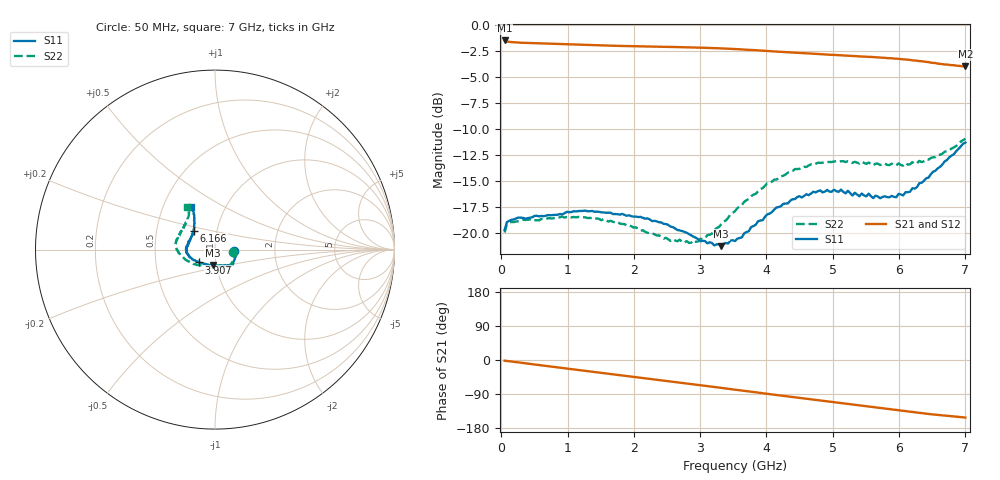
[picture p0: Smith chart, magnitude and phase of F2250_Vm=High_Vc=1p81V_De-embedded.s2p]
! Integrated Device Technology
! Corporate Headquarters
! 6024 Silver Creek Valley Road
! San Jose, CA 95138  USA
! Phone:  1-408-284-8200
! Toll Free:  1-800-223-1366
! Webpage:  http://www.idt.com/
! Timing and RF Division
! 515 Groton Road, Suite 102
! Westford, MA 01886-6024
! Device:  F2250
! Description: Voltage Variable RF Attenuator
! Frequency:  50.0 -  6000.00 MHz
! Package:  3x3 mm Thin QFN Plastic Package: 16 pin
! Ports:  2 RF, 3 DC
!  Pin  1  = GND
!  Pin  2  = NC
!  Pin  3  = RF1  = Port 1
!  Pin  4  = NC
!  Pin  5  = GND
!  Pin  6  = GND
!  Pin  7  = GND
!  Pin  8  = GND
!  Pin  9  = NC
!  Pin 10  = RF2  = Port 2
!  Pin 11  = NC
!  Pin 12  = GND
!  Pin 13  = GND
!  Pin 14  = VCNTRL
!  Pin 15  = VDD
!  Pin 16  = VMODE
! Vcntrl:  1.810 Volts
! Vmode:  +3.300 Volts
! Vdd:  +3.30  Volts
! Current:  1.324 mA
! Data:  The device was measured on a the F2250 evaluation board which has
!  individual transmission lines to the RF pins.  Data was collected
!  using a calibrated network analyzer.  The evaluation board was
!  de-embedded using a TRL calibration technique.
!  The reference plane is the edge of the package pin.
! Misc:  SN 10
!  Action Tracker AT0258
! Date Measured:  2014-11-26
! Date:  2015-10-15  MJV
! Note:
!  Integrated Device Technology supplies this data as a sample of measured
!  data at the package pin for this product.  Your particular data for this
!  product may vary.
!  Data was taken at 25 degrees C.
!  Integrated Device Technology reserves the right to change this data at anytime.
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# GHz S dB R 50
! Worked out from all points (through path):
!   201 points, 50 MHz to 7 GHz, reference 50 ohm
!   highest |S21| = -1.46 dB at 50 MHz (marker M1); lowest = -4.0 dB at 7 GHz (marker M2)
!   group delay of S21, straight-line fit = 61 ps
!   lowest |S11| = -21.2 dB at 3.317 GHz (marker M3), VSWR 1.19, Z = 48.2 - j8.35 ohm
!   |S11| at or under -10 dB: start of sweep to end of sweep
!   |S22| runs from -20.9 to -10.9 dB; largest |S21 - S12| = 0.0018
!   S11 on the Smith chart (normalised r, x): 50 MHz: 1.23, -0.02; 3.907 GHz: 0.83, -0.12; 6.166 GHz: 0.77, +0.17; 7 GHz: 0.69, +0.36
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0.05  -19.67 -5.2  -1.46 -1.9  -1.46 -1.8  -19.92 -6.5
0.08475  -18.91 -5.1  -1.57 -2.5  -1.56 -2.5  -19.11 -6.2
0.1195  -18.80 -5.9  -1.60 -3.3  -1.60 -3.3  -18.94 -6.3
0.6755  -18.29 -25.0  -1.75 -15.7  -1.75 -15.7  -18.62 -29.6
1.2315  -17.84 -40.9  -1.88 -27.9  -1.89 -27.9  -18.44 -50.9
1.75275  -18.16 -47.9  -1.98 -39.1  -1.98 -39.1  -18.88 -61.6
2.37825  -18.93 -51.2  -2.07 -52.6  -2.07 -52.6  -20.19 -72.4
2.552  -19.35 -54.5  -2.08 -56.4  -2.08 -56.4  -20.72 -78.9
2.86475  -20.18 -64.1  -2.13 -63.4  -2.13 -63.4  -20.90 -94.8
3.07325  -20.75 -76.6  -2.17 -68.1  -2.17 -68.1  -20.45 -109.2
3.3165  -21.23 -97.5  -2.23 -73.7  -2.23 -73.7  -19.15 -126.0
3.525  -20.74 -115.5  -2.29 -78.4  -2.29 -78.4  -17.87 -138.0
3.90725  -18.77 -141.4  -2.43 -87.0  -2.43 -87.0  -15.74 -156.4
4.1505  -17.51 -153.8  -2.53 -92.4  -2.53 -92.5  -14.83 -165.8
4.4285  -16.70 -163.8  -2.64 -98.5  -2.64 -98.6  -13.83 -174.5
4.7065  -16.00 -172.6  -2.73 -104.7  -2.74 -104.7  -13.40 178.8
5.1235  -15.79 176.7  -2.89 -113.9  -2.89 -113.9  -13.07 169.0
5.29725  -16.37 171.0  -2.95 -117.6  -2.95 -117.6  -13.23 165.6
5.85325  -16.53 151.3  -3.16 -129.7  -3.17 -129.8  -13.44 150.9
6.166  -15.99 138.1  -3.33 -136.6  -3.34 -136.7  -13.36 142.1
6.54825  -13.98 125.7  -3.63 -144.4  -3.64 -144.5  -12.66 129.8
7  -11.27 118.8  -3.96 -151.9  -3.97 -152.0  -10.91 122.9
